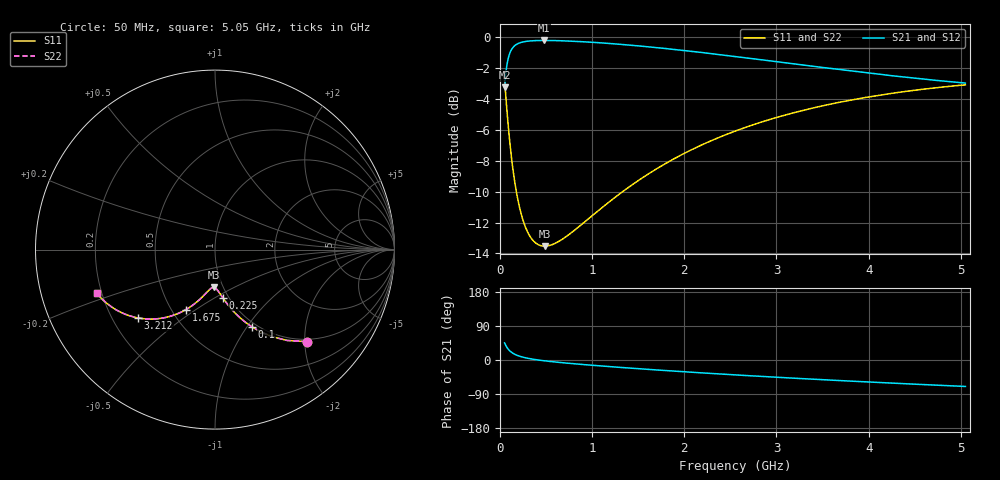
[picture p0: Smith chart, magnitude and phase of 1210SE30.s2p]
! AVX Thin Film Operation		Date: August 2001
! Description: Accu-P® Series, Thin Film, SMD, RF Capacitor
! Part Number: 12101J300FBT
! 50 MHz  -  5.05 GHz
! Serial Measurements
# mhz S db R 50
!	S11		S21		S12		S22
!	dB	Phase	dB	Phase	dB	Phase	dB	Phase
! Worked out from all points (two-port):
!   401 points, 50 MHz to 5.05 GHz, reference 50 ohm
!   highest |S21| = -0.20 dB at 475 MHz (marker M1); lowest = -3.2 dB at 50 MHz (marker M2)
!   |S21| within 3 dB of the highest: 50.61 MHz to end of sweep
!   lowest |S11| = -13.5 dB at 487.5 MHz (marker M3), VSWR 1.53, Z = 45.1 - j19.8 ohm
!   |S11| at or under -10 dB: 177.4 MHz to 1.33 GHz (1.153 GHz wide, 153 % of centre)
!   |S22| runs from -13.5 to -2.8 dB; largest |S21 - S12| = 0
!   S11 on the Smith chart (normalised r, x): 50 MHz: 0.95, -2.05; 100 MHz: 0.95, -1.06; 225 MHz: 0.94, -0.54; 1.675 GHz: 0.59, -0.46; 3.212 GHz: 0.31, -0.35; 5.05 GHz: 0.18, -0.17
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50  -2.79 -45.0  -3.24 45.0  -3.24 45.0  -2.79 -45.0
75  -4.73 -56.8  -1.78 33.2  -1.78 33.2  -4.73 -56.8
100  -6.42 -64.4  -1.13 25.6  -1.13 25.6  -6.42 -64.4
125  -7.82 -69.7  -0.79 20.3  -0.79 20.3  -7.82 -69.7
150  -8.97 -73.6  -0.59 16.4  -0.59 16.4  -8.97 -73.6
187.5  -10.33 -77.8  -0.42 12.2  -0.42 12.2  -10.33 -77.8
225  -11.34 -80.9  -0.33 9.1  -0.33 9.1  -11.34 -80.9
275  -12.28 -84.0  -0.27 5.9  -0.27 5.9  -12.28 -84.0
337.5  -13.01 -87.0  -0.22 2.9  -0.22 2.9  -13.01 -87.0
475  -13.53 -91.8  -0.20 -1.9  -0.20 -1.9  -13.53 -91.8
487.5  -13.53 -92.2  -0.20 -2.3  -0.20 -2.3  -13.53 -92.2
650  -13.18 -96.4  -0.21 -6.5  -0.21 -6.5  -13.18 -96.5
887.5  -12.12 -101.6  -0.28 -11.7  -0.28 -11.7  -12.12 -101.6
1262.5  -10.30 -108.8  -0.43 -18.8  -0.43 -18.8  -10.30 -108.8
1675  -8.61 -115.8  -0.65 -25.9  -0.65 -25.9  -8.61 -115.8
1725  -8.43 -116.7  -0.68 -26.7  -0.68 -26.7  -8.43 -116.7
2137.5  -7.11 -123.2  -0.94 -33.2  -0.94 -33.2  -7.11 -123.2
2550  -6.08 -129.3  -1.24 -39.3  -1.24 -39.3  -6.08 -129.3
3212.5  -4.84 -138.3  -1.73 -48.3  -1.73 -48.3  -4.84 -138.3
3387.5  -4.59 -140.5  -1.86 -50.6  -1.86 -50.6  -4.59 -140.5
4225  -3.65 -150.6  -2.46 -60.7  -2.46 -60.7  -3.65 -150.6
5050  -3.08 -159.8  -2.96 -69.8  -2.96 -69.8  -3.08 -159.8
